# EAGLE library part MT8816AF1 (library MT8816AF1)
Analog & Digital Crosspoint ICs Pb Free 8x16 A/log Xpt small pkg Source: Datasheet
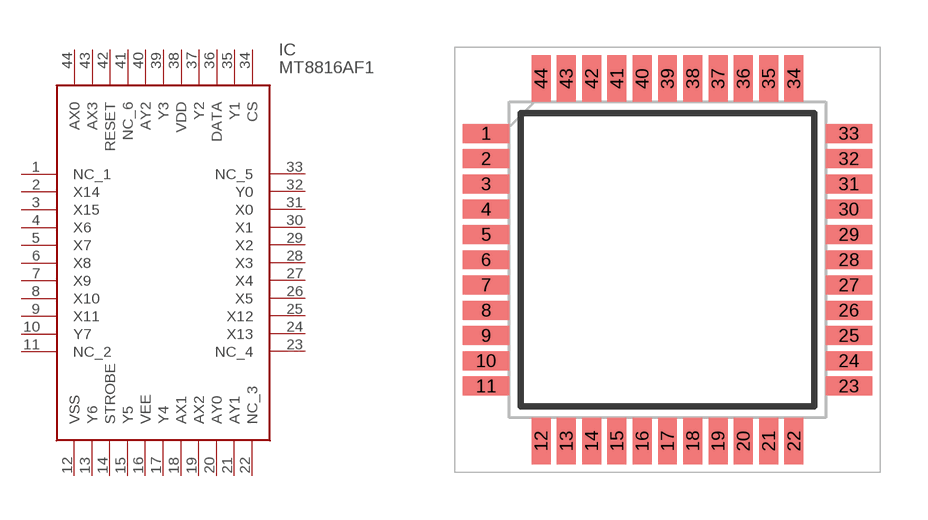
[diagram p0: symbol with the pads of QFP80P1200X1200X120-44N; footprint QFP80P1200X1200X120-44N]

Designator prefix IC

## MT8816AF1 (Description: Analog & Digital Crosspoint ICs Pb Free 8x16 A/log Xpt small pkg; Height: 1.2mm; Manufacturer_Name: Microsemi Corporation; Manufacturer_Part_Number: MT8816AF1)  [QFP80P1200X1200X120-44N]
1  NC_1
2  X14
3  X15
4  X6
5  X7
6  X8
7  X9
8  X10
9  X11
10  Y7
11  NC_2
12  VSS
13  Y6
14  STROBE
15  Y5
16  VEE
17  Y4
18  AX1
19  AX2
20  AY0
21  AY1
22  NC_3
23  NC_4
24  X13
25  X12
26  X5
27  X4
28  X3
29  X2
30  X1
31  X0
32  Y0
33  NC_5
34  CS
35  Y1
36  DATA
37  Y2
38  VDD
39  Y3
40  AY2
41  NC_6
42  RESET
43  AX3
44  AX0

## Footprint QFP80P1200X1200X120-44N (pad centres in mm)
44 Pin TQFP
smd 1.475 x 0.6: 1 -5.738,4; 2 -5.738,3.2; 3 -5.738,2.4; 4 -5.738,1.6; 5 -5.738,0.8; 6 -5.738,0; 7 -5.738,-0.8; 8 -5.738,-1.6; 9 -5.738,-2.4; 10 -5.738,-3.2; 11 -5.738,-4; 23 5.738,-4; 24 5.738,-3.2; 25 5.738,-2.4; 26 5.738,-1.6; 27 5.738,-0.8; 28 5.738,0; 29 5.738,0.8; 30 5.738,1.6; 31 5.738,2.4; 32 5.738,3.2; 33 5.738,4
smd 0.6 x 1.475: 12 -4,-5.738; 13 -3.2,-5.738; 14 -2.4,-5.738; 15 -1.6,-5.738; 16 -0.8,-5.738; 17 0,-5.738; 18 0.8,-5.738; 19 1.6,-5.738; 20 2.4,-5.738; 21 3.2,-5.738; 22 4,-5.738; 34 4,5.738; 35 3.2,5.738; 36 2.4,5.738; 37 1.6,5.738; 38 0.8,5.738; 39 0,5.738; 40 -0.8,5.738; 41 -1.6,5.738; 42 -2.4,5.738; 43 -3.2,5.738; 44 -4,5.738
